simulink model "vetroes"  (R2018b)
settings: Solver=FixedStepAuto  StartTime=0.0  StopTime=inf  RelTol=1e-3  EnableMultiTasking=on
libraries: arduinolib x3

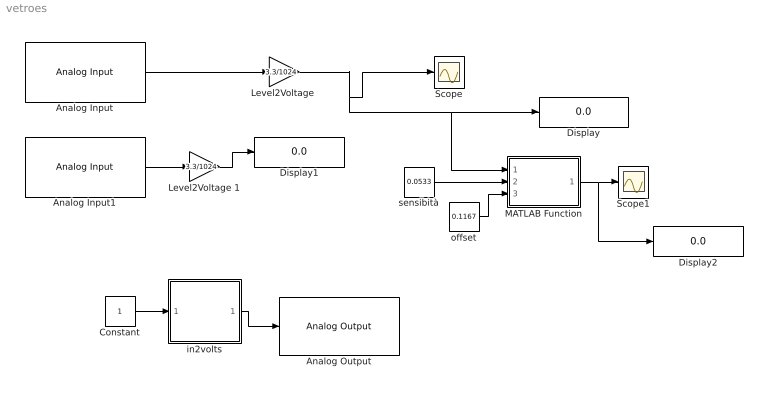
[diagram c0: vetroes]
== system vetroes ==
  Analog Input : arduinolib/Analog Input  pinNumber=0  ReadResultsOnly=off  ConversionTriggerSource=Software  ExternalTriggerType=uint32(0)  OutputDataType=uint16  EnableConversionCompleteNotify=off  EnableOuputStatus=off  SampleTime=0.1  blockPlatform=arduino
  Analog Input1 : arduinolib/Analog Input  pinNumber=1  ReadResultsOnly=off  ConversionTriggerSource=Software  ExternalTriggerType=uint32(0)  OutputDataType=uint16  EnableConversionCompleteNotify=off  EnableOuputStatus=off  SampleTime=0.1  blockPlatform=arduino
  Analog Output : arduinolib/Analog Output  DACpin=DAC0  blockPlatform=arduino
  Constant : Constant  OutDataTypeStr=int16
  Display : Display
  Display1 : Display
  Display2 : Display
  "Level2Voltage " : Gain  Gain=3.3/1024  OutDataTypeStr=double
  Level2Voltage 1 : Gain  Gain=3.3/1024  OutDataTypeStr=double
  MATLAB Function : MATLAB Function  TreatAsAtomicUnit=on
  Scope : Scope
  Scope1 : Scope
  in2volts : Subsystem
  offset : Constant  Value=0.1167  OutDataTypeStr=double
  sensibità : Constant  Value=0.0533  OutDataTypeStr=double
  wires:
  Analog Input/1 -> "Level2Voltage "/1
  in2volts/1(Out1) -> Analog Output/1
  Constant/1 -> in2volts/1(In1)
  "Level2Voltage "/1 -> MATLAB Function/1(Y), Display/1, Scope/1
  sensibità/1 -> MATLAB Function/2(s)
  offset/1 -> MATLAB Function/3(o)
  MATLAB Function/1(X) -> Display2/1, Scope1/1
  Analog Input1/1 -> Level2Voltage 1/1
  Level2Voltage 1/1 -> Display1/1

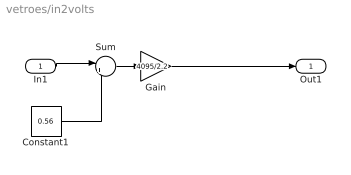
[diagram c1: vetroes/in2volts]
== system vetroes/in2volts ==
  In1 : Inport
  Constant1 : Constant  Value=0.56
  Gain : Gain  Gain=4095/2.2  OutDataTypeStr=uint16
  Sum : Sum  Inputs=|+-
  Out1 : Outport
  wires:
  Gain/1 -> Out1/1
  In1/1 -> Sum/1
  Constant1/1 -> Sum/2
  Sum/1 -> Gain/1

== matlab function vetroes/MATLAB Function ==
function X = fcn(Y,s,o)

X=(Y-o)/s;
